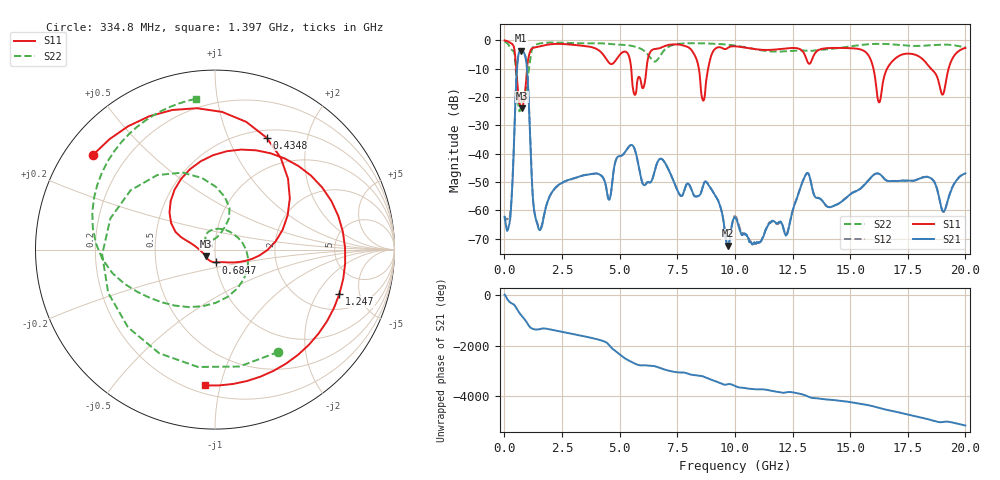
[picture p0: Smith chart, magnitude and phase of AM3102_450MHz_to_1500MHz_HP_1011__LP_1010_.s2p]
!Agilent Technologies,E8364B,MY43040894,A.07.50.67
!Agilent E8364B: A.07.50.67
!Date: Thursday, January 11, 2018 06:25:33
!Correction: S11(Full 2 Port(1,2))
!S21(Full 2 Port(1,2))
!S12(Full 2 Port(1,2))
!S22(Full 2 Port(1,2))
!S2P File: Measurements: S11, S21, S12, S22:
# Hz S  dB  R 50
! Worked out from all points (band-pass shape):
!   1601 points, 10 MHz to 20 GHz, reference 50 ohm
!   highest |S21| = -3.64 dB at 734.6 MHz (marker M1); lowest = -72.5 dB at 9.705 GHz (marker M2)
!   |S21| within 3 dB of the highest: 584.1 MHz to 933.3 MHz (349.1 MHz wide, 46 % of centre)
!   lowest |S11| = -24.1 dB at 759.6 MHz (marker M3), VSWR 1.13, Z = 45.1 - j3.37 ohm
!   |S11| at or under -10 dB: 5.502 GHz to 6.164 GHz (661.7 MHz wide, 11.3 % of centre); 16.01 GHz to 16.61 GHz (594.8 MHz wide, 3.65 % of centre); 18.5 GHz to 19.27 GHz (767.9 MHz wide, 4.07 % of centre)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
!   |S22| runs from -25.1 to -0.5 dB; largest |S21 - S12| = 0.0015
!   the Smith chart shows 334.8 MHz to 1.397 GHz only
!   S11 on the Smith chart (normalised r, x): 334.8 MHz: 0.08, +0.34; 434.8 MHz: 0.59, +1.39; 684.7 MHz: 1.00, -0.14; 1.247 GHz: 2.96, -3.18; 1.397 GHz: 0.25, -0.90
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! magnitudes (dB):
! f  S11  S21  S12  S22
! 10 MHz  -0.1  -62.3  -62.5  -0.5
! 334.8 MHz  -1.3  -52.8  -52.2  -3.5
! 434.8 MHz  -3.3  -31.5  -31.3  -4.8
! 684.7 MHz  -22.9  -3.8  -3.8  -24.6
! 734.6 MHz  -23.5  -3.6  -3.6  -22.0
! 759.6 MHz  -24.1  -3.7  -3.7  -20.9
! 984.5 MHz  -9.7  -10.3  -10.3  -15.2
! 1.247 GHz  -2.7  -56.8  -56.6  -2.4
! 1.397 GHz  -2.4  -64.2  -63.9  -1.4
! 3.346 GHz  -1.9  -47.9  -47.9  -1.1
! 4.545 GHz  -8.0  -56.3  -56.2  -1.2
! 5.657 GHz  -19.3  -38.5  -38.6  -2.2
! 6.682 GHz  -2.9  -42.4  -42.5  -6.4
! 8.081 GHz  -3.1  -52.0  -52.0  -1.0
! 8.618 GHz  -21.3  -51.4  -51.3  -1.1
! 9.705 GHz  -2.6  -72.5  -72.5  -1.6
! 10.01 GHz  -2.1  -62.6  -62.1  -1.9
! 12.23 GHz  -2.8  -68.8  -68.5  -3.9
! 13.34 GHz  -6.9  -51.8  -51.7  -3.7
! 16.68 GHz  -9.0  -49.7  -49.7  -1.4
! 19.01 GHz  -19.2  -60.3  -60.4  -1.5
! 20 GHz  -2.7  -47.0  -47.1  -2.4
